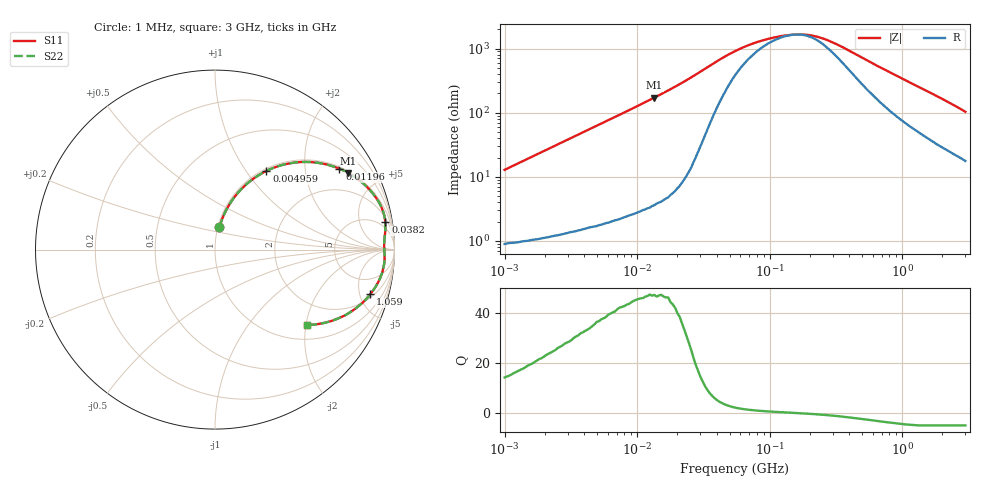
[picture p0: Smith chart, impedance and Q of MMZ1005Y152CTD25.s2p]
! S-Parameter Data Generated by TDK Corporation
! Copyright(C) 2025 TDK Corporation.
! All Rights Reserved.
! TDK P/N: MMZ1005Y152CTD25 (Chip Bead)
! Property: |Z|=1500ohm at 100MHz
! Size(LxWxT): 1x0.5x0.5mm
! Model Type: s2p (Touchstone File Format Version 1.0)
! Frequency: DC=Yes Start=1MHz Stop=3000MHz 202points Log-sweep
! Model Generated on Feb. 6, 2025
! Terms and conditions regarding TDK Simulation Models:
! 1)This simulation model is being provided solely for informational
!  purposes. Please refer to the specifications of the products in
!  terms of detailed characteristics of such products.
! 2)In no event shall TDK Corporation of any of its subsidiaries be
!  liable for any loss or damage arising, directly or indirectly,
!  from any information contained in this simulation model, including,
!  but not limited to loss or damages arising from any inaccuracies,
!  omissions or errors in connection with such information.
! 3)Any and all copyrights on this simulation model are owned by
!  TDK Corporation.  Duplication or redistribution of this simulation
!  model without prior written permission from TDK Corporation
!  is prohibited.
! 4)This simulation model is subject to any modification or change
!  without any prior notice.
! 5)Neither TDK Corporation nor any of its subsidiaries shall make any
!  warranty, express or implied, including but not limited to the
!  correctness, implied warranties of merchantability and fitness for
!  a particular purpose with respect to this simulation models.
! 6)The use of this simulation model shall be deemed to have consented
!  to the terms and conditions hereof.
! Port Assignments:
!  1 ---@@@--- 2
! Applicable Conditions:
!  Temperature = 25 degC
!  DC Bias Current = 0 A
!  Small Signal Operation
# Hz S MA R 50
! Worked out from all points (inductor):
!   201 points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, 1 MHz to 3 GHz, reference 50 ohm
!   read as one part in series: L = 2.04 uH near 1.041 MHz
!   highest Q = 47.2 at 13.49 MHz (marker M1), where L = 2.03 uH
!   self-resonance near 157.7 MHz
!   S11 on the Smith chart (normalised r, x): 1 MHz: 1.02, +0.26; 4.959 MHz: 1.03, +1.25; 11.96 MHz: 1.06, +3.03; 38.2 MHz: 3, +12; 1.059 GHz: 2.36, -6.25; 3 GHz: 1.35, -2.03
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1000000  0.1264 78.7  0.9832 -7.2  0.9832 -7.2  0.1264 78.7
2139570  0.2604 72.5  0.9546 -15.1  0.9546 -15.1  0.2604 72.5
2947212  0.3465 67.7  0.9259 -20.3  0.9259 -20.3  0.3465 67.7
3900413  0.4373 62.3  0.886 -25.9  0.886 -25.9  0.4373 62.3
4959344  0.5241 56.8  0.8374 -31.6  0.8374 -31.6  0.5241 56.8
7703107  0.6883 45.2  0.7095 -43.5  0.7095 -43.5  0.6883 45.2
1.196486e7  0.827 33.0  0.5449 -55.8  0.5449 -55.8  0.827 33.0
1.349163e7  0.8567 29.9  0.4981 -58.9  0.4981 -58.9  0.8567 29.9
1.461624e7  0.8743 27.9  0.4673 -60.9  0.4673 -60.9  0.8743 27.9
2.362996e7  0.9463 17.1  0.2941 -71.1  0.2941 -71.1  0.9463 17.1
3.820236e7  0.9611 9.1  0.1608 -71.5  0.1608 -71.5  0.9611 9.1
5.477226e7  0.9517 5.4  0.1045 -59.8  0.1045 -59.8  0.9517 5.4
7.852918e7  0.945 3.1  0.07609 -42.2  0.07609 -42.2  0.945 3.1
1.081723e8  0.9427 1.6  0.06323 -24.2  0.06323 -24.2  0.9427 1.6
1.550909e8  0.943 0.1  0.05701 -1.1  0.05701 -1.1  0.943 0.1
2.136344e8  0.9446 -1.3  0.05989 21.6  0.05989 21.6  0.9446 -1.3
3.062963e8  0.9465 -3.3  0.0773 44.6  0.0773 44.6  0.9465 -3.3
8.005644e8  0.9238 -12.0  0.2153 63.4  0.2153 63.4  0.9238 -12.0
1.059487e9  0.9011 -16.0  0.2819 61.7  0.2819 61.7  0.9011 -16.0
1.782824e9  0.8224 -25.7  0.4408 54.0  0.4408 54.0  0.8224 -25.7
2.359433e9  0.7489 -32.5  0.5458 47.5  0.5458 47.5  0.7489 -32.5
3e9  0.6635 -39.3  0.643 40.8  0.643 40.8  0.6635 -39.3
